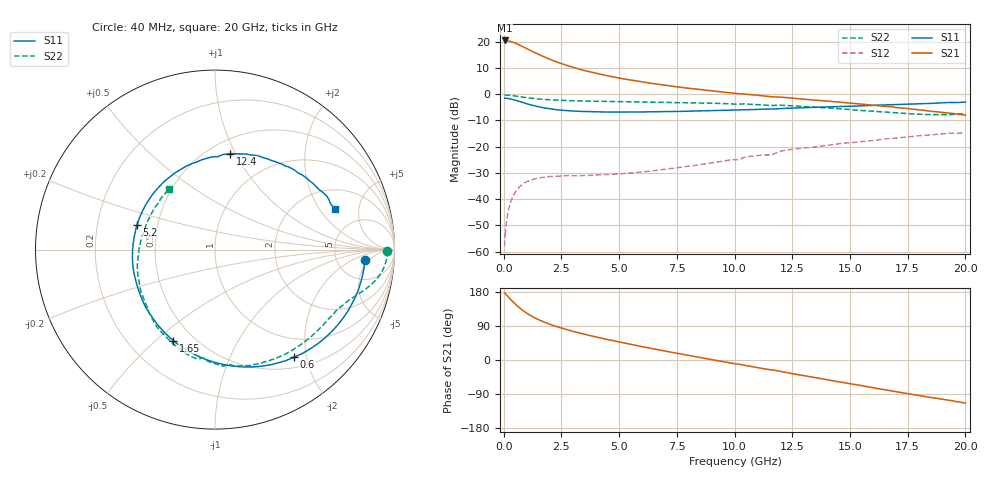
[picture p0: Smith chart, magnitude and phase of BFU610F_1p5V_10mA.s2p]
! Filename:  P:\Prog\Test\Noise\ATS_data\Testdata_Net\SplitFiles\BFU610_2W_A5_HighFreq_1.5V_10mA_D.s2p
! Date/Time: Wed 10/Aug/2011 16:54:26
! BFU610_2W_A5_HighFreq_Bias6_1.5V_1mA_10mA_R.s2p
! MDIF S-parameter v. bias file
! BFU610_2W_A5_HighFreq_1.5V_1mA_10mA
! Date/time Mon Aug 08 13:57:57 2011
! VAR V_out= 1.4999
! VAR I_out= 10.0050
! VAR V_in= 0.9422
! VAR I_in= 0.1007
! Device data file deembeded for feedlines and parallel
! Original file: \SplitFiles\BFU610_2W_A5_HighFreq_1.5V_10mA_R.s2p
! Feed-files: PR003V01_101208_Feed1.s2p, PR003V01_101208_Feed2.s2p
! Parallel-file: PR003V01_101208_Par.s2p
# MHz S MA R 50
!  Freq-MHz  S11-mag  S11-arg  S21-mag  S21-arg  S12-mag  S12-arg  S22-mag  S22-arg
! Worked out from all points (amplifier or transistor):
!   167 points, 40 MHz to 20 GHz, reference 50 ohm
!   highest |S21| = 20.4 dB at 40 MHz (marker M1)
!   |S21| within 3 dB of that: start of sweep to 974.5 MHz
!   unconditionally stable (mu >= 1): start of sweep to 41.79 MHz; 1.724 GHz to end of sweep
!   at 550 MHz: K = 0.37, MSG = 28.0 dB, |S12| = -36.7 dB
!   at 4.2 GHz: K = 2.51, MAG = 12.3 dB, |S12| = -30.7 dB
!   at 20 GHz: K = 2.78, MAG = -3.9 dB, |S12| = -14.7 dB
!   S11 on the Smith chart (normalised r, x): 40 MHz: 10, -4; 600 MHz: 0.66, -1.79; 1.65 GHz: 0.39, -0.57; 5.2 GHz: 0.38, +0.13; 12.4 GHz: 0.63, +0.95; 20 GHz: 3.11, +2.78
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40  0.8378 -3.8  10.53 177.3  0.001273 73.6  0.9591 -0.4
50  0.8353 -5.2  10.49 176.9  0.002136 75.6  0.9599 -0.7
60  0.835 -5.6  10.52 175.7  0.001929 71.7  0.9608 -0.9
140  0.8314 -13.3  10.41 170.4  0.004185 78.5  0.9585 -2.9
260  0.8161 -24.6  10.18 162.3  0.007598 74.3  0.9495 -5.4
340  0.8017 -31.8  9.927 157.2  0.009762 70.9  0.9409 -7.0
480  0.7722 -43.9  9.433 148.7  0.01318 64.7  0.923 -9.4
600  0.7445 -53.6  8.969 142.0  0.01568 59.8  0.906 -11.3
800  0.6988 -68.4  8.15 132.1  0.01902 52.5  0.8783 -13.8
1100  0.6364 -87.5  6.986 119.7  0.02246 44.2  0.8424 -16.7
1350  0.5953 -101.0  6.168 111.2  0.02437 39.1  0.819 -18.6
1650  0.5576 -114.7  5.357 102.7  0.02584 34.5  0.7976 -20.7
2000  0.5251 -128.1  4.611 94.2  0.02696 30.7  0.7802 -23.0
2400  0.5008 -141.0  3.95 86.1  0.02762 28.4  0.7617 -25.6
3400  0.4683 -165.6  2.895 69.5  0.02805 26.4  0.7405 -32.1
5200  0.4559 162.7  1.952 45.1  0.03076 31.5  0.7179 -44.7
6800  0.4623 140.8  1.516 25.8  0.03613 37.3  0.7005 -56.7
10200  0.4975 102.2  1.015 -11.4  0.0564 41.6  0.6456 -83.4
12400  0.5402 81.1  0.8474 -34.9  0.08787 33.6  0.6036 -105.0
13400  0.56 72.0  0.7734 -45.5  0.09781 26.9  0.5671 -116.0
16800  0.6286 43.6  0.5734 -81.6  0.1431 3.2  0.4472 -164.9
20000  0.7035 18.7  0.3985 -113.6  0.1836 -28.0  0.423 126.9
